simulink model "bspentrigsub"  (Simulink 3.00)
settings: Solver=ode45  SolverMode=SingleTasking  StartTime=0.0  StopTime=10.0  FixedStep=0.01  RelTol=1e-3

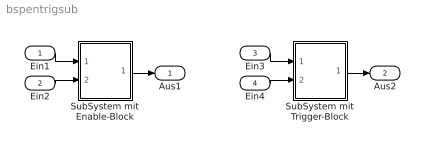
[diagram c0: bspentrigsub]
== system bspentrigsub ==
  Ein1 : Inport  Port=1  PortWidth=-1  SampleTime=-1  DataType=auto
  Ein2 : Inport  Port=2  PortWidth=-1  SampleTime=-1  DataType=auto
  Ein3 : Inport  Port=3  PortWidth=-1  SampleTime=-1  DataType=auto
  Ein4 : Inport  Port=4  PortWidth=-1  SampleTime=-1  DataType=auto
  SubSystem mit Enable-Block : Subsystem
  SubSystem mit Trigger-Block : Subsystem
  Aus1 : Outport  Port=1
  Aus2 : Outport  Port=2
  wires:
  Ein1/1 -> SubSystem mit Enable-Block/1(In1)
  Ein2/1 -> SubSystem mit Enable-Block/2(In2)
  SubSystem mit Enable-Block/1(Out1) -> Aus1/1
  Ein3/1 -> SubSystem mit Trigger-Block/1(In1)
  Ein4/1 -> SubSystem mit Trigger-Block/2(In2)
  SubSystem mit Trigger-Block/1(Out1) -> Aus2/1

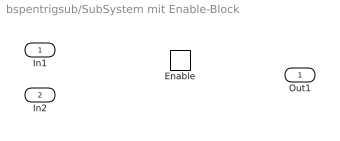
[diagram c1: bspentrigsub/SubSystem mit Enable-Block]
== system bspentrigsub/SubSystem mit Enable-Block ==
  In1 : Inport  Port=1  PortWidth=-1  SampleTime=-1  DataType=auto
  In2 : Inport  Port=2  PortWidth=-1  SampleTime=-1  DataType=auto
  Enable : EnablePort
  Out1 : Outport  Port=1

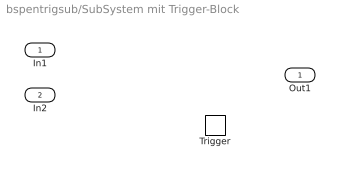
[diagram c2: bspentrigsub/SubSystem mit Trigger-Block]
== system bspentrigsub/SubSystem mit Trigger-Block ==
  In1 : Inport  Port=1  PortWidth=-1  SampleTime=-1  DataType=auto
  In2 : Inport  Port=2  PortWidth=-1  SampleTime=-1  DataType=auto
  Trigger : TriggerPort  TriggerType=rising  OutputDataType=auto
  Out1 : Outport  Port=1
